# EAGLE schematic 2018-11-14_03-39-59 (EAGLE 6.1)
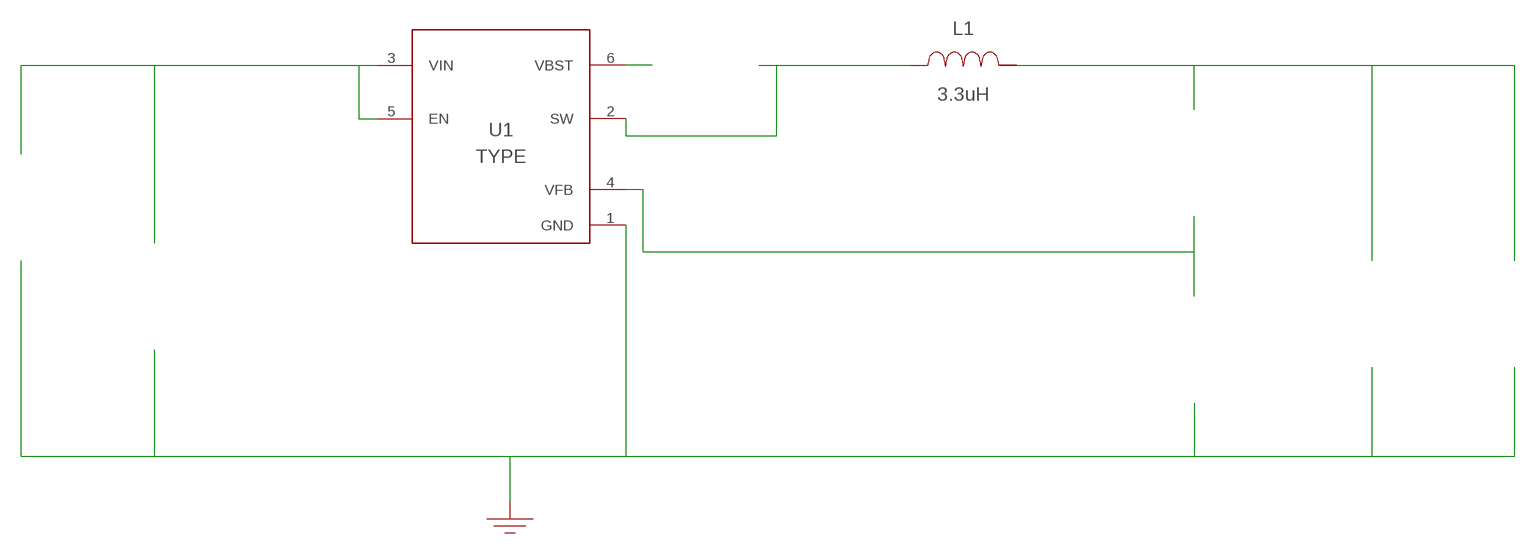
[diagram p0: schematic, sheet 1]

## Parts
CBST  100nF  C0603C104Z3VACTUC0603C104Z3VACTU  [0603]  (not placed on a sheet)
CIN  22uF  C2012X5R1V226M125ACC2012X5R1V226M125AC  [0805]  (not placed on a sheet)
COUT  47uF  JMK212BJ476MG-TJMK212BJ476MG-T  [0805]  (not placed on a sheet)
GND  WB_GND  WB_GNDWB_GND  [WB_GND]
IOUT  WB_CURRENT_LOAD  WB_CURRENT_LOADWB_CURRENT_LOAD  [WB_CURRENT_LOAD]  (not placed on a sheet)
L1  3.3uH  SDR1006-3R3MLSDR1006-3R3ML  [SDR1006]
RFBB  10k  RC0201FR-0710KLRC0201FR-0710KL  [0201]  (not placed on a sheet)
RFBT  33.2k  CRCW080533K2FKEACRCW080533K2FKEA  [0805]  (not placed on a sheet)
U1  TPS561201DDCR  TPS561201DDCRTPS561201DDCR  [DDC0006A]
VIN  WB_BATTERY  WB_BATTERYWB_BATTERY  [WB_BATTERY]  (not placed on a sheet)

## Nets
0: Cin.2@2 Cout.2@2 GND.1 Iout.-@2 Rfbb.2@2 U1.1(GND) Vin.-@2
1: Cin.1@1 U1.3(VIN) U1.5(EN) Vin.+@1
2: Cbst.1@1 L1.1 U1.2(SW)
3: Rfbb.1@1 Rfbt.2@2 U1.4(VFB)
4: Cout.1@1 Iout.+@1 L1.2 Rfbt.1@1
5: Cbst.2@2 U1.6(VBST)
Unconnected: CBST.1 CBST.2 CIN.1 CIN.2 COUT.1 COUT.2 IOUT.1(+) IOUT.2(-) RFBB.1 RFBB.2 RFBT.1 RFBT.2 VIN.1(+) VIN.2(-)

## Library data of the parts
CBST = AcceleratedDesigns_Lib:C0603C104Z3VACTU; Cap: 1.0E-7; ESR: 0.0; IRMS: 0.0; Manufacturer_Name: Kemet; Manufacturer_Part_Number: C0603C104Z3VACTU; VDC: 25.0; Vendor: Kemet
CIN = AcceleratedDesigns_Lib:C2012X5R1V226M125AC; Cap: 2.2E-5; Datasheet_URL: https://product.tdk.com/en/search/capacitor/ceramic/mlcc/info?part%5Fno%3DC2012X5R1V226M125AC; ESR: 0.00205; IRMS: 4.55587; Manufacturer_Name: TDK; Manufacturer_Part_Number: C2012X5R1V226M125AC; VDC: 35.0; Vendor: TDK
COUT = AcceleratedDesigns_Lib:JMK212BJ476MG-T; Cap: 4.7E-5; ESR: 0.0; IRMS: 0.0; Manufacturer_Name: Taiyo Yuden; Manufacturer_Part_Number: JMK212BJ476MG-T; VDC: 6.3; Vendor: Taiyo Yuden
GND = AcceleratedDesigns_Lib:WB_GND; Manufacturer_Name: WB_GND; Manufacturer_Part_Number: WB_GND; PowerPortType: POWER_GROUND; Value: Value
IOUT = AcceleratedDesigns_Lib:WB_CURRENT_LOAD; Manufacturer_Name: WB_CURRENT_LOAD; Manufacturer_Part_Number: WB_CURRENT_LOAD; PowerPortType: POWER_GROUND; Value: Value
L1 = AcceleratedDesigns_Lib:SDR1006-3R3ML; DCR: 0.024; IDC: 5.0; L: 3.3E-6; Manufacturer_Name: Bourns; Manufacturer_Part_Number: SDR1006-3R3ML; Vendor: Bourns
RFBB = AcceleratedDesigns_Lib:RC0201FR-0710KL; Datasheet_URL: http://www.yageo.com/documents/recent/PYu%2DRC%5FGroup%5F51%5FRoHS%5FL%5F5.pdf; Manufacturer_Name: Yageo; Manufacturer_Part_Number: RC0201FR-0710KL; Power: 0.05; Resistance: 10000.0; Tolerance: 1.0; Vendor: Yageo America
RFBT = AcceleratedDesigns_Lib:CRCW080533K2FKEA; Manufacturer_Name: Vishay-Dale; Manufacturer_Part_Number: CRCW080533K2FKEA; Power: 0.125; Resistance: 33200.0; Tolerance: 1.0; Vendor: Vishay-Dale
U1 = AcceleratedDesigns_Lib:TPS561201DDCR; Manufacturer: Texas Instruments; Manufacturer_Name: Texas Instruments; Manufacturer_Part_Number: TPS561201DDCR; PartNumber: TPS561201DDCR; RefDes: RefDes; TYPE: TYPE; Value: Value
VIN = AcceleratedDesigns_Lib:WB_BATTERY; Manufacturer_Name: WB_BATTERY; Manufacturer_Part_Number: WB_BATTERY; PowerPortType: POWER_GROUND; Value: Value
